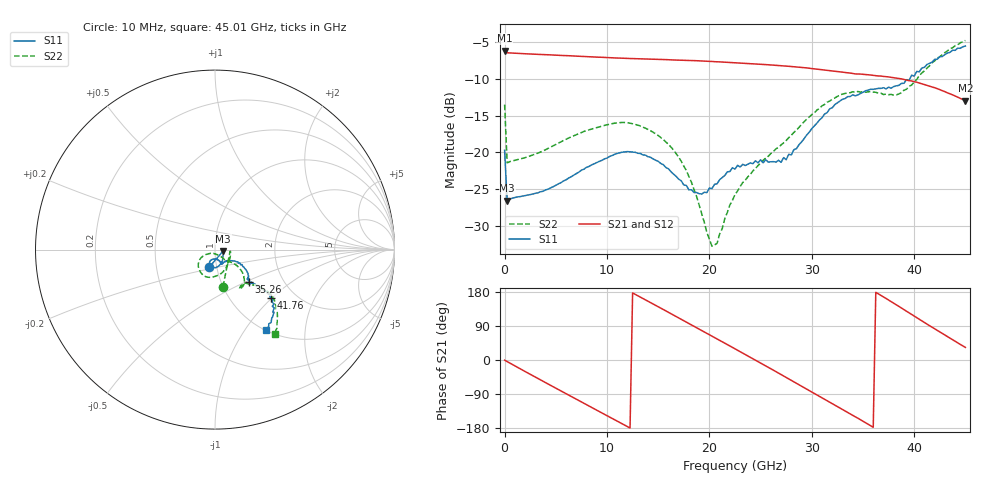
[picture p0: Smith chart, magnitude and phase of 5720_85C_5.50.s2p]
! Device:  ADRF5720
! Description: 0.5dB LSB GaAs MMIC 6-bit Digital Attenuator
! Frequency:  0.000009 -  40 GHz
! Ports:
!	RF1	= Port 1
!	RF2	= Port 2
! Vdd:  3.3 Volt
! Vss:  -3.3 Volt
! Control:  0/3.3 Volt
! State:  5.50 dB attenuation
! Data:  The device was measured using G-S-G Probes on a matrix board.
!  Data was collected using an calibrated 4 port network analyzer.
!  The reference plane for this measurement is at the launchers.
! Note:  Analog Devices supplies this data as a sample of measured data
!  for this product.  Your particular data for this product may vary.
!  Data was taken at 85 degrees C.
!  Analog Devices reserves the right to change this data at anytime.
# GHZ S DB R 45.0
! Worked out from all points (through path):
!   181 points, 10 MHz to 45.01 GHz, reference 45 ohm
!   highest |S21| = -6.14 dB at 10 MHz (marker M1); lowest = -13.0 dB at 45.01 GHz (marker M2)
!   group delay of S21, straight-line fit = 42 ps
!   lowest |S11| = -26.6 dB at 260 MHz (marker M3), VSWR 1.10, Z = 49.3 - j0.795 ohm
!   |S11| at or under -10 dB: start of sweep to 39.58 GHz
!   |S22| runs from -32.8 to -4.8 dB; largest |S21 - S12| = 0.0026
!   S11 on the Smith chart (normalised r, x): 10 MHz: 0.92, -0.18; 35.26 GHz: 1.35, -0.52; 41.76 GHz: 1.51, -0.99; 45.01 GHz: 1.01, -1.25
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0.01  -19.72 -108.3  -6.14 -0.5  -6.12 -0.4  -13.52 -77.8
0.26  -26.61 -9.9  -6.45 -4.0  -6.44 -4.0  -21.45 -6.7
2.26  -25.85 -18.8  -6.60 -34.0  -6.58 -34.0  -20.62 -23.5
4.26  -25.04 -38.1  -6.72 -63.4  -6.70 -63.3  -19.48 -46.6
7.76  -22.31 -58.5  -6.95 -114.3  -6.94 -114.3  -17.17 -76.7
11.51  -19.99 -86.7  -7.19 -168.6  -7.17 -168.5  -15.94 -107.5
13.26  -20.17 -99.7  -7.27 166.1  -7.26 166.2  -16.42 -121.7
15.26  -21.53 -110.9  -7.36 136.9  -7.34 137.1  -18.00 -137.6
17.76  -24.53 -107.0  -7.48 100.2  -7.47 100.4  -22.50 -151.3
19.01  -25.65 -91.3  -7.55 81.7  -7.53 81.8  -27.18 -148.4
20.26  -24.96 -75.8  -7.63 63.0  -7.61 63.2  -32.80 -111.6
20.76  -24.29 -72.5  -7.67 55.6  -7.65 55.8  -32.42 -85.9
22.76  -21.78 -65.7  -7.83 25.8  -7.81 26.0  -25.27 -49.7
26.01  -21.30 -57.0  -8.11 -23.1  -8.09 -22.8  -20.17 -42.8
27.51  -21.02 -44.8  -8.26 -46.0  -8.25 -45.6  -18.40 -36.6
30.26  -16.40 -30.0  -8.64 -88.2  -8.62 -88.0  -14.65 -38.4
32.51  -13.27 -34.6  -8.99 -123.0  -8.97 -122.7  -12.39 -46.8
35.26  -11.62 -43.5  -9.42 -165.6  -9.40 -165.2  -11.82 -57.2
37.76  -11.27 -41.9  -9.80 154.0  -9.78 154.4  -12.12 -51.9
39.76  -9.51 -40.3  -10.29 120.3  -10.27 120.6  -10.86 -43.5
41.76  -7.71 -41.1  -11.11 86.5  -11.09 86.9  -7.80 -39.0
45.01  -5.53 -57.7  -12.98 33.3  -12.95 33.6  -4.77 -54.7
